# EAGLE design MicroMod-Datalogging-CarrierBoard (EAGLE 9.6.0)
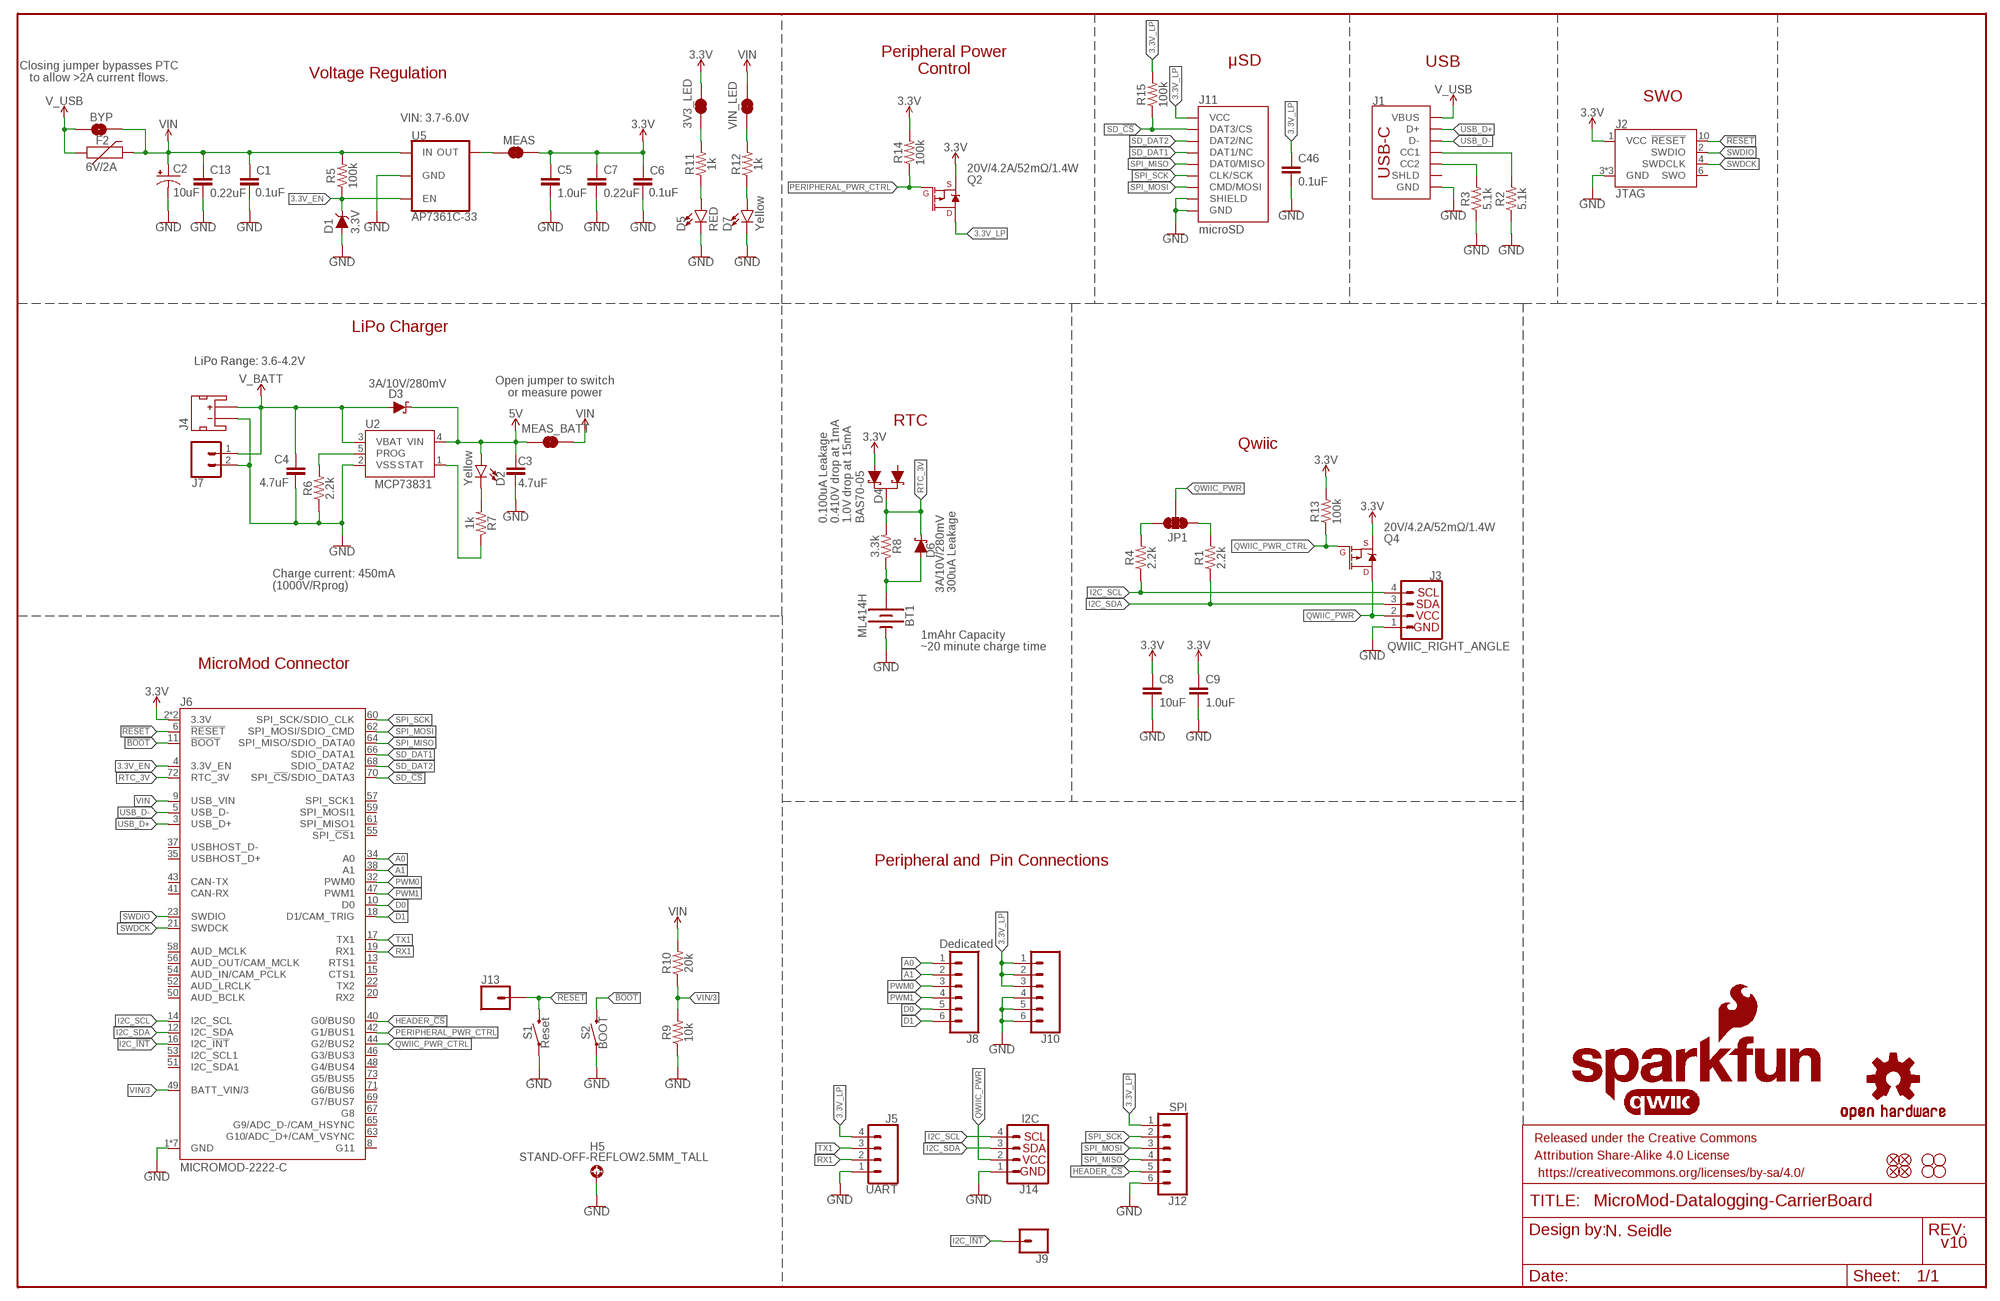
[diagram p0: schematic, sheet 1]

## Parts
3V3_LED  JUMPER-SMT_2_NC_TRACE_SILK  [SMT-JUMPER_2_NC_TRACE_SILK]
BT1  ML414H  ML414H_IV01E_BATTERY  [ML414H_IV01E]
BYP  JUMPER-SMT_2_NO_SILK  [SMT-JUMPER_2_NO_SILK]
C1  0.1uF  0.1UF-0603-25V-(+80/-20%)  [0603]
C2  10uF  10UF-POLAR-EIA3216-16V-10%(TANT)  [EIA3216]
C3  4.7uF  4.7UF-0603-35V-(20%)  [0603]
C4  4.7uF  4.7UF-0603-6.3V-(10%)  [0603]
C5  1.0uF  1.0UF-0603-16V-10%  [0603]
C6  0.1uF  0.1UF-0603-25V-(+80/-20%)  [0603]
C7  0.22uF  0.22UF-0603-25V-10%  [0603]
C8  10uF  10UF-0603-6.3V-20%  [0603]
C9  1.0uF  1.0UF-0603-16V-10%  [0603]
C13  0.22uF  0.22UF-0603-25V-10%  [0603]
C46  0.1uF  0.1UF-0603-25V-(+80/-20%)  [0603]
D1  3.3V  DIODE-ZENER-MM3Z3V3T1G  [SOD-323]
D2  Yellow  LED-YELLOW0603  [LED-0603]
D3  3A/10V/280mV  DIODE-SCHOTTKY-BAT60A  [SOD-323]
D4  BAS70-05  DIODE-SCHOTTKY-DUAL  [SOT23-3]
D5  RED  LED-RED0603  [LED-0603]
D6  3A/10V/280mV  DIODE-SCHOTTKY-BAT60A  [SOD-323]
D7  Yellow  LED-YELLOW0603  [LED-0603]
F2  6V/2A  PPTC_6V2A  [1210]
FD1  FIDUCIALUFIDUCIAL  [FIDUCIAL-MICRO]
FD2  FIDUCIALUFIDUCIAL  [FIDUCIAL-MICRO]
FD3  FIDUCIALUFIDUCIAL  [FIDUCIAL-MICRO]
FD4  FIDUCIALUFIDUCIAL  [FIDUCIAL-MICRO]
FRAME1  FRAME-LEDGER  [CREATIVE_COMMONS]
H1  STAND-OFF  [STAND-OFF]
H2  STAND-OFF  [STAND-OFF]
H3  STAND-OFF  [STAND-OFF]
H4  STAND-OFF  [STAND-OFF]
H5  STAND-OFF-REFLOW2.5MM_TALL  [STAND-OFF-REFLOW-M2.5]
J1  USB_C_2-LAYER_PADS  [USB-C-16P-2LAYER-PADS]
J2  JTAG  CORTEX_JTAG_DEBUG_MINIMUM_PTH  [2X5-PTH-1.27MM]
J3  QWIIC_RIGHT_ANGLE  QWIIC_CONNECTORJS-1MM  [JST04_1MM_RA]
J4  JST_2MM_MALE  [JST-2-SMD]
J5  UART  CONN_041X04_NO_SILK  [1X04_NO_SILK]
J6  MICROMOD-2222-C  [M.2-CONNECTOR-E]
J7  CONN_021X02_NO_SILK  [1X02_NO_SILK]
J8  Dedicated  CONN_06NO_SILK_NO_POP  [1X06_NO_SILK]
J9  CONN_01PTH_NO_SILK_YES_STOP  [1X01_NO_SILK]
J10  CONN_06NO_SILK_NO_POP  [1X06_NO_SILK]
J11  microSD  MICRO-SD-SDIOPUSH-PUSH  [MICRO-SD-SOCKET]
J12  SPI  CONN_06NO_SILK_NO_POP  [1X06_NO_SILK]
J13  CONN_01PTH_NO_SILK_YES_STOP  [1X01_NO_SILK]
J14  I2C  I2C_STANDARD_NO_SILK  [1X04_NO_SILK]
JP1  JUMPER-SMT_3_2-NC_TRACE_SILK  [SMT-JUMPER_3_2-NC_TRACE_SILK]
LOGO1  SFE_LOGO_NAME_FLAME.1_INCH  [SFE_LOGO_NAME_FLAME_.1]
LOGO2  QWIIC_LOGO_CONNECTOR  [QWIIC_5.5MM]
LOGO3  OSHW-LOGOMINI  [OSHW-LOGO-MINI]
MEAS  JUMPER-COMBO_2_NC_TRACE  [COMBO-JUMPER_2_NC_TRACE]
MEAS_BATT  JUMPER-COMBO_2_NC_TRACE  [COMBO-JUMPER_2_NC_TRACE]
Q2  20V/4.2A/52mΩ/1.4W  MOSFET_PCH-DMG2305UX-7  [SOT23-3]
Q4  20V/4.2A/52mΩ/1.4W  MOSFET_PCH-DMG2305UX-7  [SOT23-3]
R1  2.2k  2.2KOHM-0603-1/10W-1%  [0603]
R2  5.1k  5.1KOHM5.1KOHM-0603-1/10W-1%  [0603]
R3  5.1k  5.1KOHM5.1KOHM-0603-1/10W-1%  [0603]
R4  2.2k  2.2KOHM-0603-1/10W-1%  [0603]
R5  100k  100KOHM-0603-1/10W-1%  [0603]
R6  2.2k  2.2KOHM-0603-1/10W-1%  [0603]
R7  1k  1KOHM-0603-1/10W-1%  [0603]
R8  3.3k  3.3KOHM-0603-1/10W-1%  [0603]
R9  10k  10KOHM-0603-1/10W-1%  [0603]
R10  20k  20KOHM-0603-1/10W-1%  [0603]
R11  1k  1KOHM-0603-1/10W-1%  [0603]
R12  1k  1KOHM-0603-1/10W-1%  [0603]
R13  100k  100KOHM-0603-1/10W-1%  [0603]
R14  100k  100KOHM-0603-1/10W-1%  [0603]
R15  100k  100KOHM-0603-1/10W-1%  [0603]
S1  Reset  MOMENTARY-SWITCH-SPST-SMD-5.2-TALL-REDUNDANT  [TACTILE_SWITCH_SMD_5.2MM]
S2  BOOT  MOMENTARY-SWITCH-SPST-SMD-5.2-TALL-REDUNDANT  [TACTILE_SWITCH_SMD_5.2MM]
U2  MCP73831  [SOT23-5]
U5  AP7361C-33  AP7361C-33FGEUDFN-8  [UDFN-8]
VIN_LED  JUMPER-SMT_2_NC_TRACE_SILK  [SMT-JUMPER_2_NC_TRACE_SILK]

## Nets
3.3V: 3V3_LED.2 C5.1 C6.1 C7.1 C8.1 C9.1 D4.2(A1) J2.1(VCC) J6.2(3.3V) J6.74(3.3V) MEAS.2 MEAS.4 Q2.2(S) Q4.2(S) R13.2 R14.2
3.3V_EN: D1.C J6.4(3.3V_EN) R5.1 U5.5(EN)
3.3V_LP: C46.1 J5.4 J10.1 J10.2 J10.3 J11.VCC J12.1 Q2.3(D) R15.2
5V: C3.1 D2.A D3.C MEAS_BATT.1 MEAS_BATT.3 U2.4(VIN)
!BOOT!: J6.11(!BOOT!) S2.3 S2.4
!RESET!: J2.10(!RESET) J6.6(!RESET!) J13.1 S1.3 S1.4
A0: J6.34(A0) J8.1
A1: J6.38(A1) J8.2
CHG_LED: R7.1 U2.1(STAT)
D0: J6.10(D0) J8.5
D1: J6.18(D1/CAM_TRIG) J8.6
GND: BT1.- C1.2 C2.- C3.2 C4.2 C5.2 C6.2 C7.2 C8.2 C9.2 C13.2 C46.2 D1.A D5.C D7.C H5.1 J1.GND J1.GND2(GND) J2.3(GND) J2.5(GND) J2.9(GND) J3.1 J4.1(-) J5.1 J6.1(GND) J6.7(GND) J6.33(GND) J6.36(GND) J6.39(GND) J6.45(GND) J6.75(GND) J7.2 J10.4 J10.5 J10.6 J11.CD1(SHIELD) J11.GND J11.GND1(GND) J11.GND3(GND) J12.6 J14.1 R2.1 R3.1 R6.1 R9.1 S1.1 S1.2 S2.1 S2.2 U2.2(VSS) U5.4(GND) U5.EP(GND)
HEADER_!CS!: J6.40(G0/BUS0) J12.5
I2C_!INT!: J6.16(I2C_!INT!) J9.1
I2C_SCL: J3.4 J6.14(I2C_SCL) J14.4 R4.1
I2C_SDA: J3.3 J6.12(I2C_SDA) J14.3 R1.1
N$1: MEAS.1 MEAS.3 U5.1(OUT)
N$2: JP1.3 R4.2
N$3: JP1.1 R1.2
N$4: D2.C R7.2
N$5: D5.A R11.1
N$6: 3V3_LED.1 R11.2
N$7: R6.2 U2.5(PROG)
N$8: R12.2 VIN_LED.1
N$9: D7.A R12.1
N$10: J1.A5(CC1) R2.2
N$11: J1.B5(CC2) R3.2
N$14: BT1.+ D6.A R8.1
PERIPHERAL_PWR_CTRL: J6.42(G1/BUS1) Q2.1(G) R14.1
PWM0: J6.32(PWM0) J8.3
PWM1: J6.47(PWM1) J8.4
QWIIC_PWR: J3.2 J14.2 JP1.2 Q4.3(D)
QWIIC_PWR_CTRL: J6.44(G2/BUS2) Q4.1(G) R13.1
RTC_3V: D4.3(C) D6.C J6.72(RTC_3V) R8.2
RX1: J5.2 J6.19(RX1)
SD_!CS!: J6.70(SPI_!CS!/SDIO_DATA3) J11.CS(DAT3/CS) R15.1
SD_DAT1: J6.66(SDIO_DATA1) J11.RSV2(DAT1/NC)
SD_DAT2: J6.68(SDIO_DATA2) J11.RSV1(DAT2/NC)
SPI_MISO: J6.64(SPI_MISO/SDIO_DATA0) J11.DO(DAT0/MISO) J12.4
SPI_MOSI: J6.62(SPI_MOSI/SDIO_CMD) J11.DI(CMD/MOSI) J12.3
SPI_SCK: J6.60(SPI_SCK/SDIO_CLK) J11.SCLK(CLK/SCK) J12.2
SWDCK: J2.4(SWDCLK) J6.21(SWDCK)
SWDIO: J2.2(SWDIO) J6.23(SWDIO)
TX1: J5.3 J6.17(TX1)
USB_D+: J1.A6(D+) J1.B6(D+) J6.3(USB_D+)
USB_D-: J1.A7(D-) J1.B7(D-) J6.5(USB_D-)
V_BATT: C4.1 D3.A J4.2(+) J7.1 U2.3(VBAT)
V_USB: BYP.1 F2.1 J1.VBUS1(VBUS) J1.VBUS2(VBUS)
VIN: BYP.2 C1.1 C2.+ C13.1 F2.2 J6.9(USB_VIN) MEAS_BATT.2 MEAS_BATT.4 R5.2 R10.2 U5.8(IN) VIN_LED.2
VIN/3: J6.49(BATT_VIN/3) R9.2 R10.1
Unconnected: D4.1(A) J1.SHLD1(SHLD) J1.SHLD2(SHLD) J1.SHLD3(SHLD) J1.SHLD4(SHLD) J2.6(SWO) J4.NC1(PAD1) J4.NC2(PAD2) J6.8(G11) J6.13(RTS1) J6.15(CTS1) J6.20(RX2) J6.22(TX2) J6.35(USBHOST_D+) J6.37(USBHOST_D-) J6.41(CAN-RX) J6.43(CAN-TX) J6.46(G3/BUS3) J6.48(G4/BUS4) J6.50(AUD_BCLK) J6.51(I2C_SDA1) J6.52(AUD_LRCLK) J6.53(I2C_SCL1) J6.54(AUD_IN/CAM_PCLK) J6.55(SPI_!CS!1) J6.56(AUD_OUT/CAM_MCLK) J6.57(SPI_SCK1) J6.58(AUD_MCLK) J6.59(SPI_MOSI1) J6.61(SPI_MISO1) J6.63(G10/ADC_D+/CAM_VSYNC) J6.65(G9/ADC_D-/CAM_HSYNC) J6.67(G8) J6.69(G7/BUS7) J6.71(G6/BUS6) J6.73(G5/BUS5)

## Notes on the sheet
- Peripheral Power
  Control
- μSD | USB
- Closing jumper bypasses PTC
  to allow >2A current flows.
- Voltage Regulation
- SWO
- VIN: 3.7-6.0V
- LiPo Charger
- LiPo Range: 3.6-4.2V
- Open jumper to switch
  or measure power
- RTC
- Qwiic
- 0.100uA Leakage
  0.410V drop at 1mA
  1.0V drop at 15mA
- Charge current: 450mA
  (1000V/Rprog)
- 300uA Leakage
- 1mAhr Capacity
- ~20 minute charge time
- MicroMod Connector
- Peripheral and  Pin Connections
- N. Seidle
- v10

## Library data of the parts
3V3_LED VIN_LED = SparkFun-Jumpers:JUMPER-SMT_2_NC_TRACE: Normally closed trace jumper
BT1 = SparkFun-Batteries:ML414H_IV01E_BATTERY: SEIKO ML414H-IV01E Reflowable Lithium Battery; PROD_ID: BATT-14267
BYP = SparkFun-Jumpers:JUMPER-SMT_2_NO: Normally open jumper
C1 C6 C46 = SparkFun-Capacitors:0.1UF: 0.1µF ceramic capacitors; PROD_ID: CAP-00810
C2 = SparkFun-Capacitors:10UF-POLAR: 10.0µF polarized capacitors; PROD_ID: CAP-00811
C3 = SparkFun-Capacitors:4.7UF: 4.7µF ceramic capacitors; PROD_ID: CAP-14106
C4 = SparkFun-Capacitors:4.7UF: 4.7µF ceramic capacitors; PROD_ID: CAP-08280
C5 C9 = SparkFun-Capacitors:1.0UF: 1µF ceramic capacitors; PROD_ID: CAP-00868
C7 C13 = SparkFun-Capacitors:0.22UF: 0.22µF ceramic capacitors; PROD_ID: CAP-07822
C8 = SparkFun-Capacitors:10UF: 10.0µF ceramic capacitors; PROD_ID: CAP-11015
D1 = SparkFun-DiscreteSemi:DIODE-ZENER: Zener Diode; PROD_ID: DIO-11284
D2 D7 = SparkFun-LED:LED-YELLOW: Yellow SMD LED; PROD_ID: DIO-09003
D3 D6 = SparkFun-DiscreteSemi:DIODE-SCHOTTKY: Schottky diode; PROD_ID: DIO-14072
D4 = SparkFun-DiscreteSemi:DIODE-SCHOTTKY-DUAL: Diodes Incorporated - BAS70-05 Dual Schottky Diode Two Schottky Diodes in a single SOT-23 package. Low reverse current (100 nA) Vf: Datasheet referenced for footprint; PROD_ID: DIO-14829
D5 = SparkFun-LED:LED-RED: Red SMD LED; PROD_ID: DIO-00819
F2 = SparkFun-Fuses:PPTC: Resettable Fuse PPTC; PROD_ID: RES-14313
FD1-FD4 = SparkFun-Aesthetics:FIDUCIAL: Fiducial Alignment Points
FRAME1 = SparkFun-Aesthetics:FRAME-LEDGER: Schematic Frame - Ledger
H1-H4 = SparkFun-Hardware:STAND-OFF: Stand Off
H5 = SparkFun-Hardware:STAND-OFF-REFLOW: Stand Off Reflow Compatible; PROD_ID: HW-14899
J1 = SparkFun-Connectors:USB_C: USB Type C 16Pin Connector Super Speed pins not available on the 16-pin purely SMD connector so this part is best for USB 2.0 implementations. D1 and D2 are tied together enabling D+/- no matter which way the cable is plugged into the connector. The two channel configuration pins (CC1/2) are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; PROD_ID: CONN-14122
J2 = SparkFun-Connectors:CORTEX_JTAG_DEBUG_MINIMUM: Cortex Debug Connector - 10 pin Supports JTAG debug, Serial Wire debug, and Serial Wire Viewer. PTH and SMD connector options available. General Connector Information Products: PTH Connector -via Digi-Key SparkFun PSoc SparkFun T
J3 = SparkFun-Connectors:QWIIC_CONNECTOR: SparkFun I2C Standard Qwiic Connector An SMD 1mm pitch JST connector makes it easy and quick (get it? Qwiic?) to connect I2C devices to each other. The Qwiic system enables fast and solderless connection between popular platforms and various sensors and actuators. We carry 200mm, 100mm, 50mm, and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; PROD_ID: CONN-13694
J4 = SparkFun-Connectors:JST_2MM_MALE: JST 2MM MALE RA CONNECTOR Two pin, compact surface mount connector. Commonly used as a battery input connection point. We really like the solid locking feeling and high current rating on these small connectors. We use these all the time as battery connectors. Mates to single-cell LiPo batteries.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; PROD_ID: CONN-11443; SF_ID: PRT-08612
J5 = SparkFun-Connectors:CONN_04: Multi connection point. Often used as Generic Header-pin footprint for 0.1 inch spaced/style header connections On any of the 0.1 inch spaced packages, you can populate with these: Break Away Headers - Straight (PRT-00116) Break Away Male Headers - Right Angle (PRT-00553) Female Headers (PRT-00115)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; PROD_ID: CONN-09696
J6 = SparkFun-MicroMod:MICROMOD: MicroMod Connector Description: A card edge connector and mating PCB connector to allow various MicroMod Processor Boards to be coupled with various carrier boards of different capabilities. Based on the M.2 standard.; PROD_ID: CONN-14877
J7 = SparkFun-Connectors:CONN_02: Multi connection point. Often used as Generic Header-pin footprint for 0.1 inch spaced/style header connections
J8 J10 J12 = SparkFun-Connectors:CONN_06: Multi connection point. Often used as Generic Header-pin footprint for 0.1 inch spaced/style header connections On any of the 0.1 inch spaced packages, you can populate with these: Break Away Headers - Straight (PRT-00116) Break Away Male Headers - Right Angle (PRT-00553) Female Headers (PRT-00115)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
J9 J13 = SparkFun-Connectors:CONN_01: Single connection point. Often used as Generic Header-pin footprint for 0.1 inch spaced/style header connections
J11 = SparkFun-Connectors:MICRO-SD-SDIO: microSD Socket for Transflash Push-push type µSD socket. tDoc lines correctly indicate media card edge positions when inserting (unlocked, locked, depressed). NOTE: CD1 and CD2 are connected internally, and the default detect state of the socket is detect pin to ground. SparkFun Products: WAV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; PROD_ID: CONN-07820
J14 = SparkFun-Connectors:I2C_STANDARD: SparkFun I2C Standard Pinout Header SparkFun has standardized on a pinout for all I2C based sensor breakouts. This pinout allows I2C boards to be plugged directly into the headers on Arduino Uno compatible boards, and to be daisy chained easily. Example SparkFun Products: SparkFun Atmospheric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
JP1 = SparkFun-Jumpers:JUMPER-SMT_3_2-NC_TRACE: Normally closed trace jumper (2 of 2 connections) This jumper has a trace between all three pads so they are normally closed (NC). Use a razor knife to open the connection(s). For best results follow the IPC guidelines for cutting traces: Cutout at least 0.063 mm (0.005 in). Remove all loose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
LOGO1 = SparkFun-Aesthetics:SFE_LOGO_NAME_FLAME: SparkFun Font Logo w/ Flame
LOGO2 = SparkFun-Aesthetics:QWIIC_LOGO: Qwiic Logos for placement on schematic and PCB. The 5.5mm silk logo is best for placing next to Qwiic connector.
LOGO3 = SparkFun-Aesthetics:OSHW-LOGO: Open-Source Hardware (OSHW) Logo
MEAS MEAS_BATT = SparkFun-Jumpers:JUMPER-COMBO_2_NC_TRACE
Q2 Q4 = SparkFun-DiscreteSemi:MOSFET_PCH: P-channel MOSFETs Voltage controlled devices that allow control of high current outputs. SparkFun Products: SparkFun ESP32 Thing SparkFun ESP8266 Thing SparkFun Pi Servo HAT V2 DMG2305UX-7 (20V/4.2A/SOT23-3); PROD_ID: TRAN-14388
R1 R4 R6 = SparkFun-Resistors:2.2KOHM: 2.2kΩ resistor; PROD_ID: RES-08272
R2 R3 = SparkFun-Resistors:5.1KOHM; PROD_ID: RES-12083
R5 R13-R15 = SparkFun-Resistors:100KOHM: 100kΩ resistor; PROD_ID: RES-07828
R7 R11 R12 = SparkFun-Resistors:1KOHM: 1kΩ resistor; PROD_ID: RES-07856
R8 = SparkFun-Resistors:3.3KOHM: 3.3kΩ resistor; PROD_ID: RES-07851
R9 = SparkFun-Resistors:10KOHM: 10kΩ resistor; PROD_ID: RES-00824
R10 = SparkFun-Resistors:20KOHM: 20kΩ resistor; PROD_ID: RES-09383
S1 S2 = SparkFun-Switches:MOMENTARY-SWITCH-SPST: Momentary Switch (Pushbutton) - SPST; PROD_ID: SWCH-14139
U2 = SparkFun-IC-Power:MCP73831: MCP73831T Li-Ion, Li-Pol Controller Miniature single cell, fully integrated Li-Ion, Li-polymer charge management controller Datasheet SparkFun Products: SparkFun ESP32 Thing SparkFun 9DoF Razor IMU M0; PROD_ID: IC-09995
U5 = SparkFun-IC-Power:AP7361C-33FGE: AP7361C 3.3V LDO Regulator; PROD_ID: VREG-14094

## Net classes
1 power: width 0.762 mm

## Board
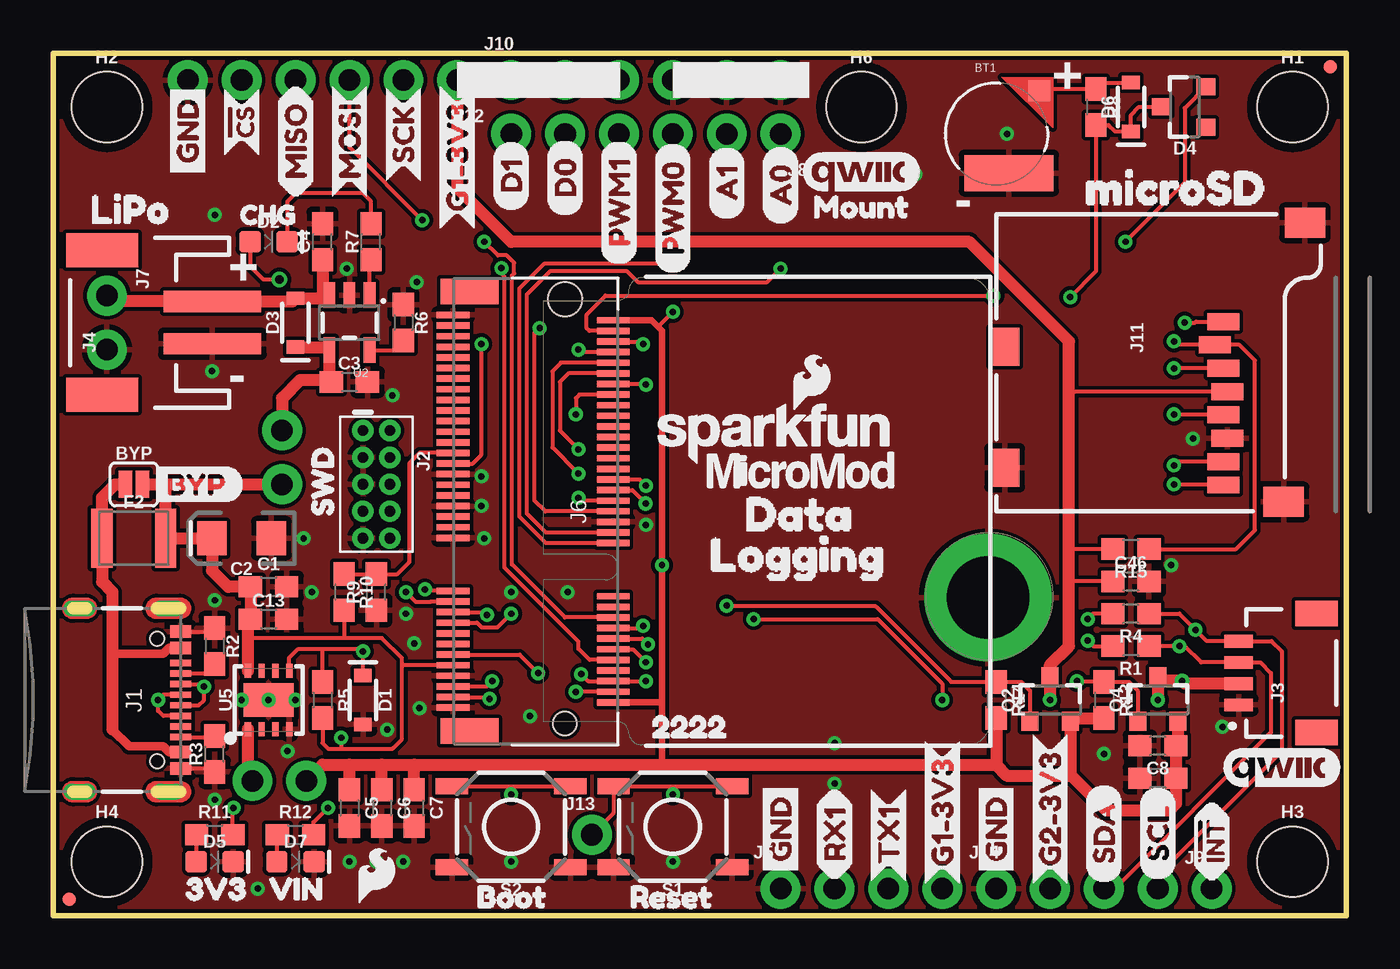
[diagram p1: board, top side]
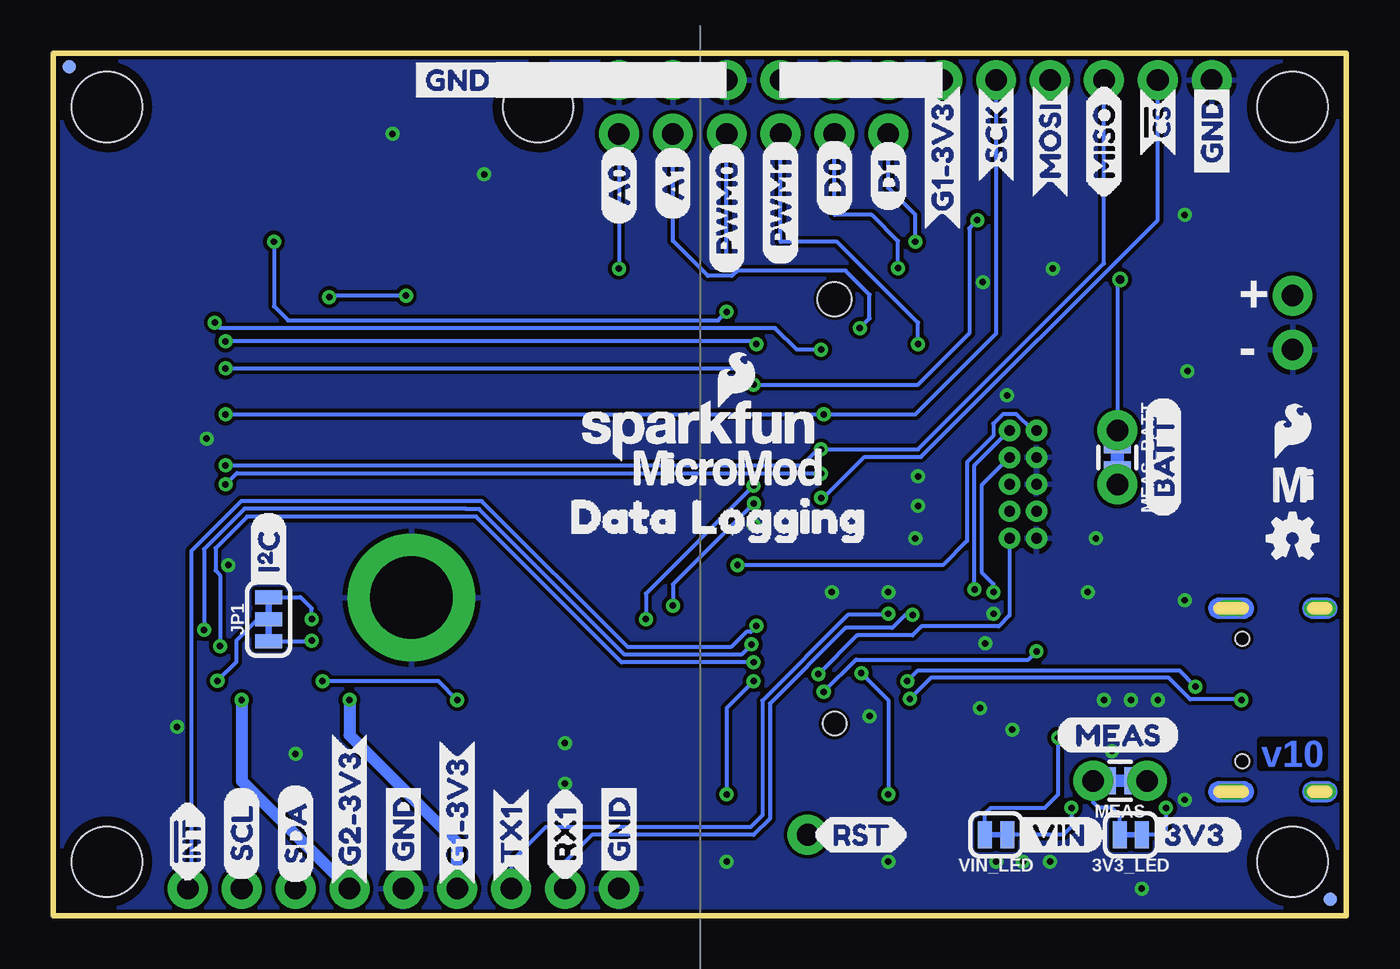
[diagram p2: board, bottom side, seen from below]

Size 60.96 x 40.64 mm. Coordinates in mm from the lower left corner, seen from the top.
Outline: 0,0 0,40.64 60.96,40.64 60.96,0 0,0
Copper layers (1*16): Top 0.035mm / dielectric 1.5mm / Bottom 0.035mm
Design rules "SparkFun-2-layer-TIGHT *": minimum track width 7mil, minimum drill 12mil, track to track 7mil, track to pad 7mil, pad to pad 7mil, via to via 7mil, smd to smd 7mil, copper to edge 7mil, drill to drill 7mil, minimum pad ring 7mil, minimum via ring 7mil, stop-mask expansion 4mil, vias tented up to drill 25mil, thermal gap 10mil

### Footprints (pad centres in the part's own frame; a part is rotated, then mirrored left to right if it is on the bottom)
SMT-JUMPER_2_NC_TRACE_SILK = smd 0.66 x 1.27: 1 -0.521,0; 2 0.521,0
ML414H_IV01E = smd 1 x 1: + 2.022,2.032 | smd 4.2 x 1.7: - 0.6,-1.85
SMT-JUMPER_2_NO_SILK = smd 0.635 x 1.27: 1 -0.406,0; 2 0.406,0
0603 = smd 1.1 x 1: 1 -0.85,0; 2 0.85,0
EIA3216 = smd 1.4 x 1.6: + 1.4,0; - -1.4,0
SOD-323 = smd 0.63 x 0.83: A 1.15,0; C -1.15,0
LED-0603 = smd 1 x 1: A -0.877,0; C 0.877,0
SOT23-3 = smd 0.8 x 0.9: 1 -0.95,-1; 2 0.95,-1; 3 0,1.1
1210 = smd 1 x 2.8: 1 -1.5,0; 2 1.5,0
FIDUCIAL-MICRO = smd 0.635 x 0.635: 1 0,0
STAND-OFF = hole 3.302: 0,0
STAND-OFF-REFLOW-M2.5 = drill 3.9 pad 6: 1 0,0
USB-C-16P-2LAYER-PADS = smd 0.3 x 1: A5 -1.25,-0.34; A6 -0.25,-0.34; A7 0.25,-0.34; A8 1.25,-0.34; B5 1.75,-0.34; B6 0.75,-0.34; B7 -0.75,-0.34; B8 -1.75,-0.34 | smd 0.6 x 1: GND -3.225,-0.34; GND2 3.225,-0.34; VBUS1 -2.45,-0.34; VBUS2 2.45,-0.34 | drill 0.4 pad 0.6 long: SHLD1 -4.318,-0.915; SHLD2 4.318,-0.915; SHLD3 -4.318,-5.095; SHLD4 4.318,-5.095 | hole 0.65: -2.89,-1.445; 2.89,-1.445
2X5-PTH-1.27MM = drill 0.508 pad 1: 1 -2.54,-0.635; 2 -2.54,0.635; 3 -1.27,-0.635; 4 -1.27,0.635; 5 0,-0.635; 6 0,0.635; 7 1.27,-0.635; 8 1.27,0.635; 9 2.54,-0.635; 10 2.54,0.635
JST04_1MM_RA = smd 0.6 x 1.35: 1 -1.5,0; 2 -0.5,0; 3 0.5,0; 4 1.5,0 | smd 1.2 x 2: NC1 2.8,-3.675; NC2 -2.8,-3.675
JST-2-SMD = smd 1 x 4.6: 1 -1,-3.7; 2 1,-3.7 | smd 1.6 x 3.4: NC1 -3.4,1.5; NC2 3.4,1.5
1X04_NO_SILK = drill 1.016 pad 1.88: 1 0,0; 2 2.54,0; 3 5.08,0; 4 7.62,0
M.2-CONNECTOR-E = smd 0.3 x 1.55: 1 9.25,-5.275; 2 9,2.275; 3 8.75,-5.275; 4 8.5,2.275; 5 8.25,-5.275; 6 8,2.275; 7 7.75,-5.275; 8 7.5,2.275; 9 7.25,-5.275; 10 7,2.275; 11 6.75,-5.275; 12 6.5,2.275; 13 6.25,-5.275; 14 6,2.275; 15 5.75,-5.275; 16 5.5,2.275; 17 5.25,-5.275; 18 5,2.275; 19 4.75,-5.275; 20 4.5,2.275; 21 4.25,-5.275; 22 4,2.275; 23 3.75,-5.275; 32 1.5,2.275; 33 1.25,-5.275; 34 1,2.275; 35 0.75,-5.275; 36 0.5,2.275; 37 0.25,-5.275; 38 0,2.275; 39 -0.25,-5.275; 40 -0.5,2.275; 41 -0.75,-5.275; 42 -1,2.275; 43 -1.25,-5.275; 44 -1.5,2.275; 45 -1.75,-5.275; 46 -2,2.275; 47 -2.25,-5.275; 48 -2.5,2.275; 49 -2.75,-5.275; 50 -3,2.275; 51 -3.25,-5.275; 52 -3.5,2.275; 53 -3.75,-5.275; 54 -4,2.275; 55 -4.25,-5.275; 56 -4.5,2.275; 57 -4.75,-5.275; 58 -5,2.275; 59 -5.25,-5.275; 60 -5.5,2.275; 61 -5.75,-5.275; 62 -6,2.275; 63 -6.25,-5.275; 64 -6.5,2.275; 65 -6.75,-5.275; 66 -7,2.275; 67 -7.25,-5.275; 68 -7.5,2.275; 69 -7.75,-5.275; 70 -8,2.275; 71 -8.25,-5.275; 72 -8.5,2.275; 73 -8.75,-5.275; 74 -9,2.275; 75 -9.25,-5.275 | smd 1.2 x 2.75: A1 10.35,-4.5; A2 -10.35,-4.5 | hole 1.1: 10,0 | hole 1.6: -10,0
1X02_NO_SILK = drill 1.016 pad 1.88: 1 0,0; 2 2.54,0
1X06_NO_SILK = drill 1.016 pad 1.88: 1 0,0; 2 2.54,0; 3 5.08,0; 4 7.62,0; 5 10.16,0; 6 12.7,0
1X01_NO_SILK = drill 1.016 pad 1.88: 1 0,0
MICRO-SD-SOCKET = smd 1.8 x 1.4: CD1 -2.05,0.4; CD2 -7.75,0.4 | smd 0.8 x 1.5: CS -7.84,10.3; DI -6.74,10.7; DO -2.34,10.7; GND -3.44,10.9; RSV1 -8.94,10.7; RSV2 -1.24,10.7; SCLK -4.54,10.7; VCC -5.64,10.9 | smd 1.4 x 1.9: GND1 -13.6,14.55; GND3 -0.45,13.55
SMT-JUMPER_3_2-NC_TRACE_SILK = smd 0.66 x 1.27: 1 -1.041,0; 2 0,0; 3 1.041,0
COMBO-JUMPER_2_NC_TRACE = smd 0.635 x 1.27: 1 -0.508,0; 2 0.508,0 | drill 1.016 pad 1.88: 3 -1.27,0; 4 1.27,0
TACTILE_SWITCH_SMD_5.2MM = smd 1.524 x 0.762: 1 -2.794,1.905; 2 2.794,1.905; 3 -2.794,-1.905; 4 2.794,-1.905
SOT23-5 = smd 0.55 x 1.2: 1 -0.95,-1.3; 2 0,-1.3; 3 0.95,-1.3; 4 0.95,1.3; 5 -0.95,1.3
UDFN-8 = smd 0.3 x 0.65: 1 -0.975,-1.375; 2 -0.325,-1.375; 3 0.325,-1.375; 4 0.975,-1.375; 5 0.975,1.375; 6 0.325,1.375; 7 -0.325,1.375; 8 -0.975,1.375 | smd 2.35 x 1.6: EP 0,0

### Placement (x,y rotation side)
3V3_LED  10.16,3.81 180 bottom
BT1  44.45,36.83 0 top
BYP  3.81,20.32 0 top
C1  10.16,15.49 0 top
C2  8.89,17.78 180 top
C3  13.97,25.15 0 top
C4  12.7,31.75 90 top
C5  13.97,5.08 270 top
C6  15.49,5.08 270 top
C7  17.02,5.08 270 top
C8  52.07,8 180 top
C9  52.07,6.48 180 top
C13  10.16,13.97 0 top
C46  50.8,15.75 0 top
D1  14.61,10.16 270 top
D2  10.16,31.75 0 top
D3  11.43,27.94 90 top
D4  53.34,38.1 90 top
D5  7.62,2.54 0 top
D6  50.8,38.1 90 top
D7  11.43,2.54 0 top
F2  3.81,17.78 0 top
FD1  0.76,0.76 0 top
FD2  60.2,40.01 0 top
FD3  0.76,0.76 0 bottom
FD4  60.2,40.01 0 bottom
FRAME1  not placed on the board
H1  58.42,38.1 0 top
H2  2.54,38.1 0 top
H3  58.42,2.54 0 top
H4  2.54,2.54 0 top
H5  44.07,14.99 0 top
H6  STAND-OFF  [STAND-OFF]  38.1,38.1 0 top
J1  6.35,10.16 270 top
J2  15.24,20.32 270 top
J3  55.88,11.43 90 top
J4  3.81,27.94 90 top
J5  34.29,1.27 0 top
J6  24.13,19.05 270 top
J7  2.54,29.21 270 top
J8  34.29,36.83 180 top
J9  54.61,1.27 0 top
J10  21.59,39.37 0 top
J11  44.45,19.05 270 top
J12  19.05,39.37 180 top
J13  25.4,3.81 0 top
J14  44.45,1.27 0 top
JP1  50.8,13.97 90 bottom
LOGO1  34.04,22.73 0 top
LOGO2  57.91,6.99 0 top
LOGO3  2.54,17.78 0 bottom
LOGO4  SFE_LOGO_NAME_FLAME.1_INCH  [SFE_LOGO_NAME_FLAME_.1]  30.48,22.86 0 bottom
LOGO5  QWIIC_LOGO_CONNECTOR  [QWIIC_5.5MM]  38.1,35.05 0 top
MEAS  10.67,6.35 180 bottom
MEAS_BATT  10.79,21.59 270 bottom
Q2  46.99,10.16 0 top
Q4  52.07,10.16 0 top
R1  50.8,12.7 180 top
R2  7.62,12.7 270 top
R3  7.62,7.62 90 top
R4  50.8,14.22 180 top
R5  12.7,10.16 270 top
R6  16.51,27.94 270 top
R7  14.99,31.75 90 top
R8  49.15,38.1 270 top
R9  15.24,15.24 90 top
R10  13.72,15.24 270 top
R11  7.62,3.81 0 top
R12  11.43,3.81 0 top
R13  49.53,10.16 270 top
R14  44.45,10.16 270 top
R15  50.8,17.27 180 top
S1  29.21,4.19 180 top
S2  21.59,4.19 180 top
U2  13.97,27.94 180 top
U5  10.16,10.16 0 top
U$1  [SFE_LOGO_FLAME_.1]  2.54,22.86 0 bottom
U$2  [RESET3]  26.29,0.89 0 top
U$3  [G1#3V32]  19.05,32.26 90 top
U$4  [DATA3]  37.97,18.8 0 bottom
U$5  [MEAS]  13.72,8.51 0 bottom
U$6  [GND_P]  6.35,34.54 90 top
U$7  [MOSI_O]  13.97,33.78 90 top
U$8  [MISO_I]  11.43,33.78 90 top
U$9  [SCK_O]  16.51,34.54 90 top
U$10  [!CS_O]  8.89,35.56 90 top
U$11  [MOUNT2]  34.92,33.4 0 top
U$12  [D13]  21.59,33.15 90 top
U$13  [D13]  21.59,33.15 90 bottom
U$14  [D02]  24.13,32.89 90 top
U$15  [PWM10]  26.67,30.61 90 top
U$16  [D02]  24.13,32.89 90 bottom
U$17  [G1#3V32]  41.91,1.4 90 bottom
U$18  [CHG2]  8,33.02 0 top
U$19  [BOOT2]  19.05,0.89 0 top
U$20  [3V3_TO]  5.33,1.27 0 top
U$21  [!INT_I]  54.61,1.4 90 top
U$22  [LOGGING4]  32.51,18.8 0 bottom
U$23  [G1#3V32]  19.05,32.26 90 bottom
U$24  [SWD3]  12.7,17.91 90 top
U$25  [RX10]  36.83,1.65 90 bottom
U$26  [VIN_TO]  9.27,1.27 0 top
U$27  [BYP0]  4.45,20.32 0 top
U$28  [MICROSD4]  47.24,34.29 0 top
U$29  [RX10]  36.83,1.65 90 top
U$30  [DATA3]  31.24,18.92 0 top
U$31  [TX13]  39.37,1.52 90 top
U$32  [GND_P]  34.29,1.65 90 top
U$33  [LIPO0]  0.64,33.27 0 top
U$34  [LOGGING4]  29.34,17.02 0 top
U$35  [!INT_I]  54.61,1.4 90 bottom
U$36  [GND_P]  44.45,1.65 90 top
U$37  [MICROMOD_LOGO_.35]  29.21,21.08 0 bottom
U$38  [G2#3V31]  46.99,1.4 90 bottom
U$39  [SDA_IO]  49.53,1.52 90 top
U$40  [SCL_IO]  52.07,1.65 90 top
U$41  [TX13]  39.37,1.52 90 bottom
U$42  [GND_P]  34.29,1.65 90 bottom
U$43  [A00]  34.29,32.51 90 top
U$44  [A00]  34.29,32.51 90 bottom
U$45  [GND_P]  44.45,1.65 90 bottom
U$46  [3V31]  9.53,3.81 0 bottom
U$47  [SDA_IO]  49.53,1.52 90 bottom
U$48  [SCL_IO]  52.07,1.65 90 bottom
U$49  [SCK_O]  16.51,34.54 90 bottom
U$50  [MOSI_O]  13.97,33.78 90 bottom
U$51  [MISO_I]  11.43,33.78 90 bottom
U$52  [!CS_O]  8.89,35.56 90 bottom
U$53  [GND_P]  6.35,34.54 90 bottom
U$54  [GND_P]  44.32,39.37 0 bottom
U$55  [22229]  27.3,8.89 0 top
U$56  [I#C0]  50.8,15.24 90 bottom
U$57  [A10]  31.75,32.77 90 top
U$58  [A10]  31.75,32.77 90 bottom
U$59  [PWM01]  29.21,30.23 90 top
U$60  [PWM01]  29.21,30.23 90 bottom
U$61  [PWM10]  26.67,30.61 90 bottom
U$62  [MICROMOD_MI_LOGO_.35]  2.54,20.32 0 bottom
U$63  [MICROMOD_LOGO_.35]  35.18,20.95 0 top
U$66  [SFE_LOGO_FLAME_.1]  15.24,1.91 0 top
U$67  [VIN0]  15.75,3.81 0 bottom
U$68  [RST_I]  25.15,3.81 0 bottom
U$69  [G1#3V32]  41.91,1.4 90 top
U$70  [G2#3V31]  46.99,1.4 90 top
U$71  [BATT1]  8.64,18.8 90 bottom
VIN_LED  16.51,3.81 180 bottom

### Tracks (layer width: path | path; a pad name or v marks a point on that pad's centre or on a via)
3.3V  (via drill 0.3)
  Top 0.178: v29.21,28.45 28.51,27.75 | D4.2 53.34,38.05 53.34,34.54 v50.55,31.75
  Top 0.305: 28.7,10.03 28.7,7.11 | 28.7,10.03 v28.7,16.51 28.7,27.56 28.51,27.75 28.21,28.05 J6.74 | 28.7,10.03 28.68,10.05 J6.2
  Top 0.559: 44.43,7.11 44.94,6.6 48.01,6.6 | 13.97,7.11 12.7,7.11 MEAS.4 | 13.97,7.11 15.49,7.11 | 15.49,7.11 17.02,7.11 | 17.02,7.11 28.7,7.11 44.43,7.11 | 48.01,6.6 47.94,6.67 Q2.2 48.09,9.31 R13.2 | 44.43,7.11 44.45,7.13 R14.2 | C5.1 13.97,7.11 | C6.1 15.49,7.11 | C7.1 17.02,7.11 | Q4.2 53.02,8.1 C8.1 C9.1 52.92,5.29 52.58,4.95 49.66,4.95 48.01,6.6
  Bottom 0.178: MEAS.2 MEAS.4 11.94,5.33 11.68,5.08 11.05,5.08 10.68,4.71 3V3_LED.2 | v50.55,31.75 50.55,28.7 49.89,28.04 29.62,28.04 v29.21,28.45 | J2.1 14.79,22.86 15.56,23.63 16.19,23.63 16.64,23.18 16.64,22.6 17.88,21.36 17.88,17.65 19.02,16.51 v28.7,16.51
3.3V_EN  (via drill 0.3)
  Top 0.178: U5.5 11.13,12.15 11.56,12.57 12.7,12.57 | 12.7,12.57 14.48,12.57 v14.61,12.45 D1.C | R5.1 12.7,12.57 | J6.4 v24.64,10.54
  Bottom 0.178: v14.61,12.45 14.99,12.06 23.11,12.06 v24.64,10.54
3.3V_LP  (via drill 0.3)
  Top 0.178: J11.VCC 47.93,24.69 47.88,24.64 | R15.2 47.88,17.27 | C46.1 47.88,15.75
  Top 0.559: v46.99,10.16 Q2.3 46.99,11.81 47.88,12.7 47.88,15.75 47.88,17.27 47.88,24.64 47.88,27.05 43.18,31.75 21.59,31.75 19.05,34.29 J12.1 J10.1 J10.2 J10.3
  Bottom 0.559: J5.4 41.91,3.43 46.99,8.51 v46.99,10.16
5V  (via drill 0.38)
  Top 0.178: D2.A 9.28,30.59 9.91,29.97 v10.67,29.97
  Top 0.559: D3.C 12.87,26.79 U2.4 13.02,25.25 | 13.02,25.25 C3.1 | 13.02,25.25 11.66,25.25 10.79,24.38 MEAS_BATT.3
  Bottom 0.178: MEAS_BATT.1 MEAS_BATT.3 10.79,29.84 v10.67,29.97
!BOOT!  (via drill 0.3)
  Top 0.178: v22.86,11.43 21.99,12.3 J6.11 | S2.4 21.59,6.1 | 21.59,6.1 S2.3 | v21.59,5.71 21.59,6.1
  Bottom 0.178: v22.86,11.43 21.59,10.16 v21.59,5.71
!RESET!  (via drill 0.3)
  Top 0.178: v27.94,11.05 J6.6 25.22,11.05 v24.89,11.38 | 29.21,6.1 S1.4 26.42,4.83 J13.1 | 29.21,6.1 S1.3 | v29.21,5.71 29.21,6.1
  Bottom 0.178: v27.94,11.05 29.21,9.78 v29.21,5.71 | J2.10 15.88,14.14 16.39,13.63 20.03,13.63 20.45,13.21 23.06,13.21 v24.89,11.38
A0  (via drill 0.3)
  Top 0.178: v34.29,30.48 33.66,29.84 27.56,29.84 27.03,30.38 23.44,30.38 22.34,29.27 22.34,18.94 23.23,18.05 J6.34
  Bottom 0.178: J8.1 v34.29,30.48
A1  (via drill 0.3)
  Top 0.178: v22.93,27.69 22.69,27.45 22.69,19.56 23.2,19.05 J6.38
  Bottom 0.178: J8.2 31.75,31.8 30.09,30.14 28.96,30.14 28.71,30.39 23.61,30.39 22.48,29.26 22.48,28.14 v22.93,27.69
CHG_LED
  Top 0.178: U2.1 14.92,30.83 R7.1
D0  (via drill 0.3)
  Top 0.178: v21.13,30.51 21.13,30.25 21.27,30.11 21.27,16.4 24.77,12.91 24.77,12.57 25.29,12.05 J6.10
  Bottom 0.178: v21.13,30.51 21.13,31.78 22.38,33.02 24.13,33.02 J8.5
D1  (via drill 0.3)
  Top 0.178: v20.32,31.75 20.96,31.11 21.38,31.11 21.73,30.75 21.73,30.26 21.63,30.16 21.63,16.55 24.13,14.05 J6.18
  Bottom 0.178: v20.32,31.75 20.32,33.02 21.59,34.29 J8.6
GND  (via drill 0.3)
  Top 0.178: J1.GND 7.46,13.38 R2.1 | J1.GND2 7.46,6.93 R3.1
  other vias: 7.62,5.46 11.05,7.75 10.16,10.16 11.43,10.16 8.89,10.16 15.75,8.76 17.27,9.78 13.97,2.54 15.24,2.54 16.51,2.54 16.64,14.22 12.19,15.24 11.81,17.78 7.62,14.86 17.14,29.84 7.49,25.65 7.62,33.02 27.94,18.41 20.19,19.3 20.19,20.7 20.32,17.78 55.12,8.89 53.72,22.48 52.7,16.51 40.64,34.92 49.53,7.62 24.26,15.24 21.59,15.24 36.83,8.13 36.83,6.22 29.21,2.54 21.59,2.54 9.65,1.27 44.96,36.83 17.02,12.83 22.48,9.4 13.84,30.48 16,24.51
  pour Bottom (isolate 0.178): 0,40.64 60.96,40.64 60.96,0 0,0
  pour Top (isolate 0.178): 0,40.64 60.96,40.64 60.96,0 0,0
HEADER_!CS!  (via drill 0.3)
  Top 0.178: J6.40 24.9,19.55 v24.77,19.68
  Bottom 0.178: J12.5 8.89,32.77 20.05,21.61 22.71,21.61 24.64,19.68 v24.77,19.68
I2C_!INT!  (via drill 0.3)
  Top 0.178: J6.16 27.72,13.55 v27.81,13.65
  Bottom 0.178: v27.81,13.65 28.09,13.37 28.29,13.37 29.01,12.65 33.87,12.65 40.75,19.53 52.09,19.53 54.45,17.17 54.45,1.44 J9.1
I2C_SCL  (via drill 0.3)
  Top 0.178: J14.4 52.07,1.91 57.91,7.75 57.91,12.45 57.43,12.93 J3.4 54.38,12.93 v53.85,13.46 53.09,14.22 R4.1 | J6.14 27.77,13.05 v28.04,12.78
  Bottom 0.178: v28.04,12.78 28.52,12.29 34.02,12.29 40.87,19.15 41.5,19.15 41.53,19.18 51.94,19.18 53.85,17.27 v53.85,13.46
I2C_SDA  (via drill 0.3)
  Top 0.178: J14.3 50.04,1.27 57.4,8.64 57.4,11.43 56.9,11.93 J3.3 54.11,11.93 53.34,12.7 v53.09,12.7 R1.1 | J6.12 27.33,12.55 v27.94,11.94
  Bottom 0.178: v27.94,11.94 34.16,11.94 41.02,18.8 51.82,18.8 53.3,17.31 53.3,16.26 53.09,16.05 v53.09,12.7
N$1
  Top 0.559: U5.1 9.19,6.56 MEAS.3
  Bottom 0.178: MEAS.3 MEAS.1
N$2  (via drill 0.3)
  Top 0.178: R4.2 49.02,14.22 v48.77,13.97
  Bottom 0.178: JP1.3 49.3,15.01 48.77,14.48 v48.77,13.97
N$3  (via drill 0.3)
  Top 0.178: v48.77,12.95 49.02,12.7 R1.2
  Bottom 0.178: JP1.1 48.79,12.93 v48.77,12.95
N$4
  Top 0.178: 14.99,32.37 R7.2 14.99,33.66 14.61,34.04 11.43,34.04 11.04,33.64 D2.C
N$5
  Top 0.178: R11.1 6.74,3.78 D5.A
N$6  (via drill 0.3)
  Top 0.178: R11.2 8.47,5.04 v8.51,5.08
  Bottom 0.178: v8.51,5.08 8.51,4.06 8.76,3.81 3V3_LED.1
N$7
  Top 0.178: U2.5 16.06,26.64 R6.2
N$8  (via drill 0.3)
  Top 0.178: R12.2 12.28,4.41 v12.95,5.08
  Bottom 0.178: v12.95,5.08 12.95,4.19 13.34,3.81 VIN_LED.1
N$9
  Top 0.178: R12.1 10.55,3.78 D7.A
N$10
  Top 0.178: J1.A5 7.18,11.41 R2.2
N$11
  Top 0.178: J1.B5 7.56,8.41 R3.2
N$14
  Top 0.178: BT1.+ 46.56,38.95 R8.1 49.45,39.25 D6.A
PERIPHERAL_PWR_CTRL  (via drill 0.3)
  Top 0.178: J6.42 27.3,20.05 v27.93,19.42 | v31.75,14.61 31.79,14.57 38.77,14.57 42.33,11.01 R14.1 45.63,11.01 46.04,10.6 Q2.1
  Bottom 0.178: v27.93,19.42 31.75,15.6 v31.75,14.61
PWM0  (via drill 0.3)
  Top 0.178: v29.21,30.73 23.17,30.73 21.98,29.55 21.98,18.8 23.23,17.55 J6.32
  Bottom 0.178: v29.21,30.73 J8.3
PWM1  (via drill 0.3)
  Top 0.178: v20.19,26.92 20.19,21.72 19.78,21.3 J6.47
  Bottom 0.178: v20.19,26.92 20.19,27.94 24,31.75 26.67,31.75 J8.4
QWIIC_PWR  (via drill 0.3)
  Top 0.559: J3.2 53.34,10.93 v53.21,11.06 52.27,11.06 Q4.3 v52.07,10.16
  Bottom 0.178: JP1.2 51.31,13.97 52.32,12.95 52.32,11.95 v53.21,11.06
  Bottom 0.559: v52.07,10.16 52.07,6.35 J14.2
QWIIC_PWR_CTRL  (via drill 0.3)
  Top 0.178: J6.44 27.65,20.55 v27.94,20.26 | v33.02,13.97 38.87,13.97 41.91,10.93 v41.91,10.16 | v48.26,11.05 49.49,11.05 R13.1 50.71,11.01 51.12,10.6 Q4.1
  Bottom 0.178: v27.94,20.26 33.02,15.18 v33.02,13.97 | v41.91,10.16 42.8,11.05 v48.26,11.05
RTC_3V  (via drill 0.3)
  Top 0.178: v44.32,29.21 26.04,29.21 25.15,28.32 25.15,27.69 25.28,27.55 J6.72 | v47.94,29.15 49.15,30.35 R8.2 49.74,37.25 50.05,36.95 D6.C 50.8,37.72 51.18,38.1 D4.3
  Bottom 0.178: v44.32,29.21 47.88,29.21 v47.94,29.15
RX1  (via drill 0.3)
  Top 0.178: v20.45,14.17 20.32,14.3 J6.19
  Bottom 0.178: v20.45,14.17 20.8,14.17 21.41,13.56 23.6,13.56 27.18,9.99 27.18,4.57 27.94,3.81 35.56,3.81 36.83,2.54 J5.2
SD_!CS!  (via drill 0.3)
  Top 0.178: v27.81,26.92 27.69,27.05 J6.70 | v52.83,27.05 52.99,26.89 J11.CS 55.91,26.89 56.64,26.16 56.64,18.16 55.75,17.27 R15.1
  Bottom 0.178: v27.81,26.92 27.94,27.05 v52.83,27.05
SD_DAT1  (via drill 0.3)
  Top 0.178: J11.RSV2 52.86,20.29 v52.83,20.32 | J6.66 23.94,26.05 23.53,25.65 23.53,22.06 v24.77,20.83
  Bottom 0.178: v24.77,20.83 24.79,20.85 52.3,20.85 v52.83,20.32
SD_DAT2  (via drill 0.3)
  Top 0.178: v53.34,27.94 53.83,27.94 53.88,27.99 J11.RSV1 | v24.77,26.67 24.77,26.55 J6.68
  Bottom 0.178: v24.77,26.67 25.91,26.67 26.92,27.69 53.09,27.69 v53.34,27.94
SPI_MISO  (via drill 0.3)
  Top 0.178: J11.DO 53.01,21.39 v52.83,21.21 | J6.64 24.29,25.55 23.89,25.15 23.89,22.85 v24.77,21.97
  Bottom 0.178: J12.4 11.43,30.73 20.19,21.97 v24.77,21.97 24.83,22.04 25.65,21.21 v52.83,21.21
SPI_MOSI  (via drill 0.3)
  Top 0.178: J11.DI 52.84,25.79 v52.83,25.78 | v27.94,25.02 27.91,25.05 J6.62 | J12.3 13.97,36.2 v17.4,32.77
  Bottom 0.178: v52.83,25.78 28.7,25.78 v27.94,25.02 20.19,25.02 17.78,27.43 17.78,32.38 v17.4,32.77
SPI_SCK  (via drill 0.3)
  Top 0.178: J11.SCLK 52.86,23.59 v52.83,23.62 | J6.60 24.8,24.55 24.64,24.38 v24.64,23.62
  Bottom 0.178: J12.2 16.51,27.43 20.32,23.62 v24.64,23.62 v52.83,23.62
SWDCK  (via drill 0.3)
  Top 0.178: J6.21 17.8,14.8 17.77,14.77 17.11,14.77 v16.64,15.24
  Bottom 0.178: v16.64,15.24 16.64,15.62 17.17,16.15 17.17,20.3 J2.4
SWDIO  (via drill 0.3)
  Top 0.178: J6.23 17.59,15.3 v17.53,15.37
  Bottom 0.178: v17.53,15.37 17.53,21.21 J2.2
TX1  (via drill 0.3)
  Top 0.178: v21.59,14.22 20.94,13.58 20.2,13.58 19.98,13.8 J6.17
  Bottom 0.178: v21.59,14.22 21.64,14.17 23.5,14.17 27.53,10.13 27.53,4.72 28.09,4.17 37.74,4.17 39.37,2.54 J5.3
USB_D+  (via drill 0.3)
  Top 0.178: J1.A6 5.2,10.41 v4.95,10.16 4.95,9.65 5.2,9.41 J1.B6 | v20.57,10.21 20.48,10.3 J6.3
  Bottom 0.178: v4.95,10.16 4.99,10.2 7.36,10.2 8.36,11.2 19.59,11.2 v20.57,10.21
USB_D-  (via drill 0.3)
  Top 0.178: J1.B7 6.99,10.91 v7.11,10.79 7.11,10.16 6.86,9.91 J1.A7 | v20.7,11.05 20.45,10.8 J6.5
  Bottom 0.178: v20.7,11.05 20.2,11.55 7.87,11.55 v7.11,10.79
V_BATT
  Top 0.559: J7.1 2.81,28.94 J4.2 11.28,28.94 D3.A 12.57,29.09 | 12.57,29.09 12.87,29.09 U2.3 | C4.1 12.7,29.22 12.57,29.09
V_USB
  Top 0.406: J1.VBUS2 5.46,7.71 5.2,7.98 3.58,7.98 2.79,8.76 | J1.VBUS1 5.46,12.61 5.2,12.34 2.95,12.34 2.79,12.19
  Top 0.559: BYP.1 2.92,20.32 2.31,19.71 F2.1 2.31,15.72 2.79,15.24 2.79,12.19 2.79,8.76
VIN  (via drill 0.3)
  Top 0.178: 13.72,13.08 15.49,13.08 16.45,12.13 16.45,11.81 | 13.72,13.08 9.19,13.08 | R10.2 13.72,13.08 | R5.2 12.7,8.13 12.95,7.87 13.59,7.87 | 13.59,7.87 16,7.87 16.45,8.32 16.45,11.81 | 16.45,11.81 16.46,11.8 J6.9 | v13.59,8.38 13.59,7.87
  Top 0.559: BYP.2 5.33,20.32 | 5.33,20.32 5.31,20.3 F2.2 C2.+ 7.49,16.26 8.26,15.49 C1.1 C13.1 9.19,13.85 9.19,13.08 U5.8 | 5.33,20.32 MEAS_BATT.4
  Bottom 0.178: MEAS_BATT.2 MEAS_BATT.4 | VIN_LED.2 17.03,4.81 16.76,5.08 14.22,5.08 13.59,5.71 v13.59,8.38
VIN/3
  Top 0.178: R10.1 R9.2 16.22,16.09 16.79,16.66 16.79,21.31 17.27,21.8 J6.49

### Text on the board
Bottom: v10
tPlace: + | - | + | -
bPlace: + | -
tDocu: N. Seidle

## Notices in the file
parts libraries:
SparkFun-Aesthetics: Licensing: Creative Commons ShareAlike 4.0 International - https://creativecommons.org/licenses/by-sa/4.0
SparkFun-Aesthetics: Released under the Creative Commons Attribution Share-Alike 4.0 License
SparkFun-Aesthetics: https://creativecommons.org/licenses/by-sa/4.0
